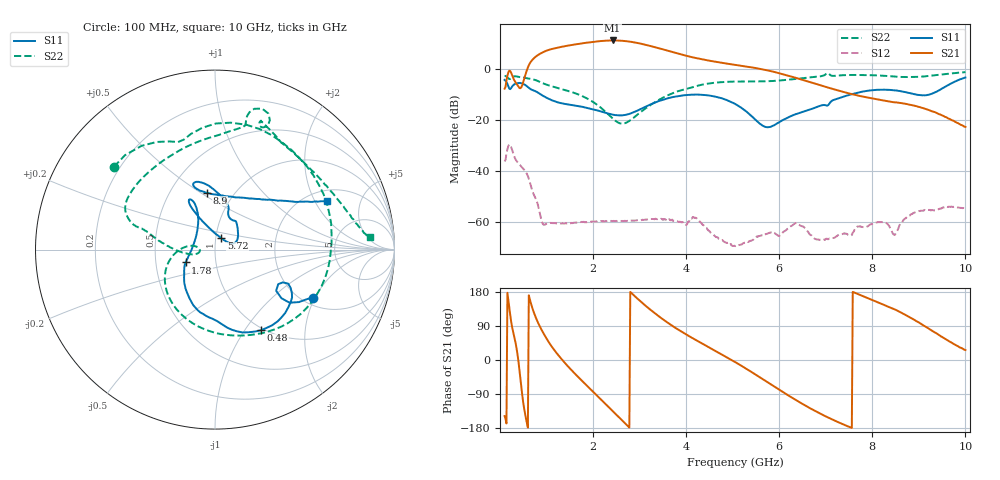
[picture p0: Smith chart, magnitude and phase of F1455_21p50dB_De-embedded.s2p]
! Integrated Device Technology
! Corporate Headquarters
! 6024 Silver Creek Valley Road
! San Jose, CA 95138  USA
! Phone:  1-408-284-8200
! Toll Free:  1-800-223-1366
! Webpage:  http://www.idt.com/
! Timing and RF Division
! 515 Groton Road, Suite 102
! Westford, MA 01886-6024
! Device:  F1455
! Description: 6-bit 0.5 dB Transmit Variable Gain Amplifier
! Frequency:  1400.0 -  2300.00 MHz
! Package:  6x6 mm Thin QFN Plastic Package: 28 pin
! State:  43
! Atten State:  21.5 dB
! Voltage:  +5.00 Volts
! Current:  217.607 mA
! Data:  The device was measured on a the F1455 evaluation board which has
!  individual transmission lines to the RF pins.  Data was collected
!  using a calibrated network analyzer.  The evaluation board was
!  de-embedded using a TRL calibration technique.
!  The reference plane is the edge of the package pin.
!  Pin  1 = CSb
!  Pin  2 = DATA
!  Pin  3 = CLK
!  Pin  4 = RSET
!  Pin  5 = GND
!  Pin  6 = RFIN  = Port 1
!  Pin  7 = GND
!  Pin  8 = NC
!  Pin  9 = NC
!  Pin 10 = NC
!  Pin 11 = NC
!  Pin 12 = NC
!  Pin 13 = NC
!  Pin 14 = /STBY
!  Pin 15 = GND
!  Pin 16 = RFOUT  = Port 2
!  Pin 17 = GND
!  Pin 18 = NC
!  Pin 19 = NC
!  Pin 20 = NC
!  Pin 21 = GND
!  Pin 22 = NC
!  Pin 23 = GND
!  Pin 24 = NC
!  Pin 25 = NC
!  Pin 26 = NC
!  Pin 27 = GND
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# GHz S dB R 50
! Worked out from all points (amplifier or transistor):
!   496 points, 100 MHz to 10 GHz, reference 50 ohm
!   highest |S21| = 11.2 dB at 2.42 GHz (marker M1)
!   |S21| within 3 dB of that: 1.196 GHz to 3.402 GHz (2.206 GHz wide, 95.9 % of centre)
!   unconditionally stable (mu >= 1): start of sweep to end of sweep
!   at 1.74 GHz: K = 141.36, MAG = 10.5 dB, |S12| = -60.1 dB
!   at 5.06 GHz: K = 820.99, MAG = 3.5 dB, |S12| = -69.6 dB
!   at 10 GHz: K = 511.32, MAG = -14.1 dB, |S12| = -54.8 dB
!   S11 on the Smith chart (normalised r, x): 100 MHz: 2.26, -1.93; 480 MHz: 0.97, -1.19; 1.78 GHz: 0.71, -0.11; 5.72 GHz: 1.06, +0.13; 8.9 GHz: 0.75, +0.53; 10 GHz: 2.47, +2.51
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0.1  -4.32 -26.2  -7.74 -148.1  -36.35 47.2  -2.76 140.7
0.18  -6.76 -36.2  -1.37 159.4  -30.25 -7.2  -3.70 112.7
0.26  -6.93 -25.0  -2.42 87.6  -31.79 -76.9  -3.32 95.9
0.38  -5.56 -42.1  -6.54 12.2  -36.73 -117.2  -3.04 57.9
0.48  -5.72 -60.2  -6.30 -93.4  -38.77 -148.7  -3.33 32.0
0.68  -8.14 -90.2  3.22 143.3  -46.99 138.7  -3.96 -14.2
0.96  -10.92 -123.4  6.89 65.1  -61.22 127.1  -5.90 -70.5
1.34  -13.53 -144.8  8.76 -0.0  -60.64 103.2  -7.98 -121.0
1.76  -14.84 -155.9  10.04 -54.7  -60.08 71.9  -10.59 -158.0
1.78  -14.94 -156.4  10.10 -57.1  -60.15 71.2  -10.76 -159.5
2.12  -16.43 -166.2  10.88 -98.1  -59.90 53.8  -14.53 178.5
2.42  -17.93 175.7  11.19 -134.6  -59.77 42.2  -19.43 170.7
2.82  -17.40 138.9  10.65 177.2  -59.58 31.1  -19.91 -167.8
3.1  -15.10 122.2  9.61 146.1  -59.27 24.4  -15.92 -172.5
3.4  -12.73 115.0  8.20 116.6  -58.86 12.4  -12.33 177.8
4.1  -10.12 116.2  4.74 60.3  -58.62 -3.5  -7.39 164.0
5.06  -13.81 116.6  1.61 -6.0  -69.63 -5.4  -4.95 148.9
5.72  -22.85 60.7  -0.45 -56.4  -64.81 9.7  -4.84 121.6
6.7  -15.69 39.2  -5.36 -129.8  -65.51 -128.8  -3.24 78.8
8.36  -8.22 107.9  -12.79 139.8  -61.60 83.6  -2.82 62.8
8.9  -9.89 98.2  -14.42 106.0  -56.46 110.2  -3.16 41.4
10  -3.36 23.7  -22.76 26.3  -54.76 29.9  -1.27 4.7
